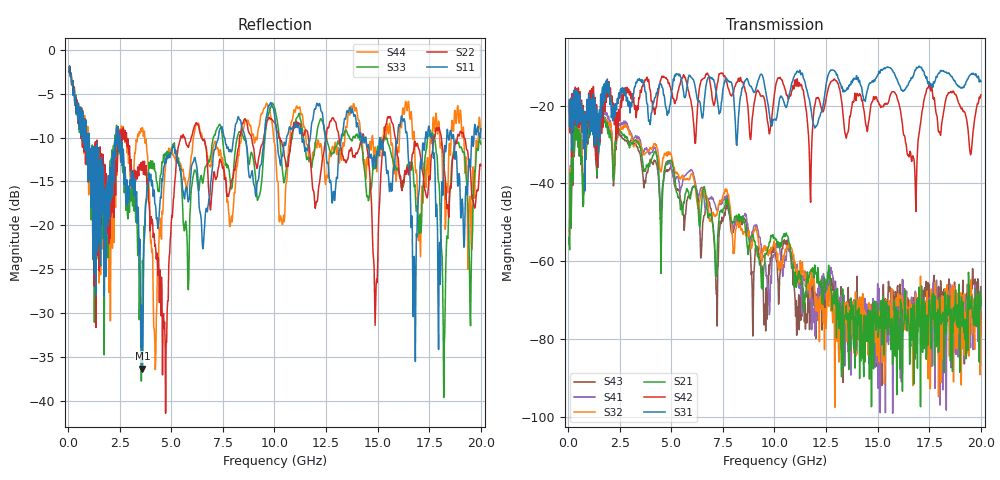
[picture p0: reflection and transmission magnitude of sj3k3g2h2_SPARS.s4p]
! FILE: E:\users\goganessyan\GBX_Backplane\FR408_backplane\1m_OUTBOUND_FEXT\sj3k3g2h2_SPARS.s4p
# MHZ S RI R 50.00
! FREQ  S11  S12  S13  S14
!  S21  S22  S23  S24
!  S31  S32  S33  S34
!  S41  S42  S43  S44
!  REAL  IMAG  REAL  IMAG  REAL  IMAG  REAL  IMAG
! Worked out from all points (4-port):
!   799 points, 50 MHz to 20 GHz, reference 50 ohm
!   strongest paths, dB at 50 MHz, 5.025 GHz, 10.03 GHz, 15.03 GHz, 20 GHz:
!     S31: -18.5, -16.1, -23.4, -11.9, -13.8
!     S42: -19.1, -16.6, -16.1, -18.9, -17.2
!     S21: -53.9, -34.4, -54.2, -79.6, -71.4
!     S32: -52.4, -33.2, -55.5, -76.7, -79.4
!     S41: -52.1, -36.4, -57.5, -92.8, -67.9
!     S43: -55.8, -36.8, -57.5, -70.7, -66.6
!   lowest |S11| = -36.3 dB at 3.6 GHz (marker M1), VSWR 1.03, Z = 50.6 - j1.42 ohm
!   |S11| at or under -10 dB: 1.027 GHz to 2.321 GHz (1.294 GHz wide, 77.3 % of centre); 2.514 GHz to 7.282 GHz (4.768 GHz wide, 97.3 % of centre); 8.577 GHz to 9.51 GHz (932.4 MHz wide, 10.3 % of centre)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
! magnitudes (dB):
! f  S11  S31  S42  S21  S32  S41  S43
! 50 MHz  -2.5  -18.5  -19.1  -53.9  -52.4  -52.1  -55.8
! 425 MHz  -6.1  -16.1  -15.6  -25.5  -23.0  -22.9  -25.2
! 3.6 GHz  -36.3  -13.4  -14.9  -33.8  -31.9  -31.4  -36.9
! 4.225 GHz  -17.6  -17.9  -21.1  -31.9  -29.8  -30.9  -34.2
! 13.25 GHz  -9.6  -15.5  -18.7  -89.7  -80.4  -80.3  -74.1
! 18.23 GHz  -12.0  -11.3  -20.5  -88.7  -72.1  -75.6  -67.1
! 20 GHz  -9.0  -13.8  -17.2  -71.4  -79.4  -67.9  -66.6
